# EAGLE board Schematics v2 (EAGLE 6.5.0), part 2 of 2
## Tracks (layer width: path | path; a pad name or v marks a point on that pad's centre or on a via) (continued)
N$201  (via drill 0.5) (continued)
  Bottom 0.813: C117.2 C118.2 23.76,93.34 23.24,93.34 22.73,93.85 v22.73,94.23
N$202
  Top 0.813: C120.1 35.84,91.09 33.53,88.77 19.18,88.77 18.54,88.14 18.54,86.79 U$7.P$6
N$203
  Top 0.813: C121.1 35.84,93.37 32.38,89.92 17.65,89.92 16.64,88.9 16.64,86.67 U$7.P$5
N$204
  Top 0.813: C120.2 38.94,88.29 R41.1
N$205
  Top 0.813: R42.1 36.7,96.19 C121.2
N$206
  Bottom 0.813: X9.1 6.41,88.52 8,90.04 10.79,90.04 12.06,88.77 21.43,88.77 C106.1
N$207
  Top 0.406: U$7.P$30 5.69,97.31 JP8.1
N$208
  Top 0.406: U$7.P$1 9.5,87.59 8.32,88.77 7.62,88.77 6.99,89.41 6.99,94.11 6.03,95.06 4.13,95.06 2.98,96.2 2.98,97.09 JP8.2
N$209
  Bottom 0.813: X9.3 6.03,93.6 7.62,92.33 11.81,92.33 12.32,91.82 21.46,91.82 C105.1
N$210
  Bottom 0.813: U$7.P$29 11.28,95.46 L7.1
N$211
  Bottom 0.813: C122.2 63.27,8.48 62.1,9.65 62.1,10.92 61.34,11.68 60.83,11.68 60.33,12.19 60.33,13.54 U$8.P$11 U$8.P$12 U$8.P$13 U$8.P$14
N$212
  Bottom 0.813: C123.2 63.79,13.45 U$8.P$9 | U$8.P$7 U$8.P$8 U$8.P$9 | U$8.P$9 U$8.P$10
N$213
  Bottom 0.813: C124.1 54.14,11.39 53.21,12.32 U$8.P$15
N$214
  Bottom 0.813: U$8.P$16 53.24,4.34 53.98,5.08 53.98,8.6 C124.2
N$215
  Bottom 0.813: U$8.P$17 55.02,4.47 55.24,4.7 55.24,8 55.63,8.38 55.88,8.38 56.26,8.76 56.26,11.05 56.64,11.43 58.61,11.43 C125.1
N$216
  Bottom 0.813: C125.2 57.9,9.64 57.4,9.14 57.4,8.38 56.64,7.62 56.64,3.05 U$8.P$18
N$217
  Bottom 0.813: U$8.P$27 72.8,4.79 C126.1
N$218
  Bottom 0.813: U$8.P$26 71.02,5.07 C127.1
N$219
  Bottom 0.813: U$8.P$25 69.24,5.07 C128.1
N$220
  Bottom 0.813: U$8.P$23 65.68,5.07 C129.1
N$221
  Bottom 0.813: U$8.P$24 67.46,5.07 C130.1
N$222
  Bottom 0.813: U$8.P$28 74.57,5.04 C131.1
N$223
  Bottom 0.813: U$8.P$19 58.57,5.07 C132.1
N$224
  Bottom 0.813: U$8.P$20 60.35,5.07 C133.1
N$225
  Bottom 0.813: U$8.P$21 62.13,5.07 C134.1
N$226
  Bottom 0.813: U$8.P$22 63.91,5.07 C135.1
N$227  (via drill 0.5)
  Top 0.813: C136.1 81.05,13.43 v80.42,12.8 | v77.37,11.4 76.33,12.45 U$8.P$2
  Bottom 0.813: v80.42,12.8 79.5,11.81 79.1,11.4 v77.37,11.4
N$228  (via drill 0.5)
  Top 0.813: R43.1 70.77,7.28 v72.01,5.97
  Bottom 0.813: C128.2 C127.2 70.98,6.86 71.5,6.86 71.88,6.48 v72.01,5.97
N$229  (via drill 0.5)
  Top 0.813: R44.1 67.15,7.28 v68.45,5.97
  Bottom 0.813: C129.2 C130.2 67.42,6.86 67.94,6.86 68.45,6.35 v68.45,5.97
N$230  (via drill 0.5)
  Top 0.813: v61.34,6.03 60.33,7.11 59.75,7.11 R45.2
  Bottom 0.813: C133.2 C132.2 60.57,6.87 v61.34,6.03
N$231  (via drill 0.5)
  Top 0.813: R46.2 63.59,7.28 v64.9,5.97
  Bottom 0.813: C134.2 C135.2 63.87,6.86 64.39,6.86 64.9,6.35 v64.9,5.97
N$232
  Top 0.813: C137.1 51.79,9.12 54.1,11.43 68.45,11.43 69.09,12.06 69.09,13.41 U$8.P$6
N$233
  Top 0.813: C138.1 51.79,6.84 55.24,10.29 69.98,10.29 70.99,11.3 70.99,13.54 U$8.P$5
N$234
  Top 0.813: C137.2 50.47,11.92 R47.1
N$235
  Top 0.813: R48.1 50.93,4.01 C138.2
N$236
  Bottom 0.813: X10.1 81.22,11.68 79.63,10.16 76.83,10.16 75.56,11.43 66.2,11.43 C123.1
N$237
  Top 0.406: U$8.P$30 81.94,2.9 JP9.1
N$238
  Top 0.406: U$8.P$1 78.13,12.61 79.31,11.43 80.01,11.43 80.64,10.79 80.64,6.1 81.6,5.14 83.5,5.14 84.64,4 84.64,3.11 JP9.2
N$239
  Bottom 0.813: X10.3 81.6,6.6 80.01,7.87 75.82,7.87 75.31,8.38 66.17,8.38 C122.1
N$240
  Bottom 0.813: U$8.P$29 76.35,4.74 L8.1
N$241  (via drill 0.5)
  Top 0.61: IC2.1 82.8,41.91 82.17,41.27 v81.03,41.27 | 78.28,46.79 78.28,47.19 77.98,47.5 | v77.6,44.83 77.6,46.23 78.22,46.85
  Top 1.016: C140.2 77.98,47.5 77.98,47.09 78.22,46.85 78.28,46.79 R50.2
  Bottom 0.61: v81.03,41.27 80.26,41.27 78.36,43.18 78.36,44.07 v77.6,44.83
N$242
  Bottom 0.61: IC5.2 IC5.1 87.12,85.79 C192.1
N$243
  Bottom 0.61: C193.1 84.84,83.57 84.07,82.8 IC5.6 IC5.7
N$244  (via drill 0.5)
  Top 0.406: IC2.7 81.53,36.47 R51.2
  Top 0.61: IC2.7 81.53,36.32 82.17,35.69 v82.17,34.04 | v73.15,51.05 73.15,51.31 72.01,52.45 72.01,63.63 72.64,64.26 72.64,65.53 73.28,66.17 77.47,66.17 C142.2
  Bottom 0.61: v82.17,34.04 82.17,39.37 81.66,39.88 81.66,40.39 82.04,40.77 82.04,45.47 81.41,46.1 79.12,46.1 76.83,48.39 73.79,48.39 73.15,49.02 v73.15,51.05
N$245
  Top 0.406: U$10.1 78.61,52.45 C140.1
N$246
  Top 0.61: U$10.8 78.61,62.23 C142.1
N$247
  Top 0.406: U$10.2 79.88,52.58 C141.1
N$248
  Top 0.61: U$10.7 79.88,62.35 C143.1
N$249
  Bottom 0.305: U3.3 43.33,53.09 R52.2
N$250  (via drill 0.5)
  Top 0.254: RN2.5 76.74,26.57 77.32,27.15 77.32,29.18 77.06,29.44 74.02,29.44 73.51,28.93 73.51,27.41 73.25,27.15 71.98,27.15 71.22,26.39 70.46,26.39 69.95,25.88 52.68,25.88 JP1.2
  Top 0.305: v78.03,24.61 77.16,24.61 RN2.5
  Bottom 0.305: U1.20 78.28,24.56 v78.03,24.61
N$251  (via drill 0.5)
  Top 0.254: 76.05,25.14 76.05,26.77 76.43,27.15 v76.43,28.55 76.05,28.93 74.27,28.93 74.02,28.68 74.02,26.9 73.76,26.64 72.24,26.64 71.48,25.88 70.71,25.88 70.21,25.38 53.44,25.38 52.43,24.36 JP1.4
  Top 0.305: 76.05,25.14 RN2.6
  Bottom 0.254: U1.18 76.99,27.99 v76.43,28.55
N$252  (via drill 0.5)
  Top 0.254: v74.85,27.94 74.85,26.14 | 74.85,26.14 75.16,25.83 75.16,25.27 RN2.7 | 74.85,26.14 72.49,26.14 71.73,25.38 70.97,25.38 70.46,24.87 55.98,24.87 54.97,23.85 JP1.6
  Bottom 0.254: U1.16 75.69,27.08 v74.85,27.94
N$253  (via drill 0.5)
  Top 0.254: RN2.8 73.92,24.61 v72.24,24.61 71.48,24.61 71.22,24.36 58.01,24.36 57.51,23.85 JP1.8
  Bottom 0.254: U1.14 74.4,25.25 74.02,24.87 72.49,24.87 v72.24,24.61
N$254  (via drill 0.5)
  Top 0.254: JP1.10 61.32,21.82 61.32,19.28 62.08,18.52 68.94,18.52 69.57,19.15 70.84,19.15 71.22,19.53 72.24,19.53 72.75,20.04 v72.75,20.8 73.09,21.14 RN1.5
  Bottom 0.254: U1.11 74.4,21.18 74.02,21.57 73.51,21.57 v72.75,20.8
N$255  (via drill 0.5)
  Top 0.254: RN1.6 75.29,21.04 75.29,20.55 75.54,20.3 75.54,20.04 76.05,19.53 v76.05,18.44 75.39,17.75 70.08,17.75 69.06,16.74 64.62,16.74 v63.86,17.5 | JP1.12 62.59,22.58 63.86,21.31 v63.86,19.41
  Bottom 0.254: v63.86,19.41 v63.86,17.5 | U1.9 75.69,19.25 76.05,18.9
  Bottom 0.305: 76.05,18.9 v76.05,18.44
N$256  (via drill 0.5)
  Top 0.254: v77.6,17.78 77.6,18.75 76.05,20.55 76.05,21 RN1.7 | JP1.14 65.13,22.84 66.37,21.59 71.25,21.59 72.11,22.45 v72.11,22.84
  Bottom 0.254: v72.11,22.84 72.87,22.07 76.56,22.07 | 77.06,20.24 U1.7 | 76.81,21.57 77.06,21.31 77.06,20.24 | 77.06,20.24 77.06,19.35 77.49,18.87 77.49,17.86
  Bottom 0.305: 76.56,22.07 76.81,21.82 76.81,21.57 | 77.49,17.86 v77.6,17.78
N$257
  Bottom 1.016: C192.2 87.12,95.25 X11.1
N$258  (via drill 0.5)
  Top 0.406: v47.24,48.26 v47.24,52.45
  Bottom 0.305: v47.24,52.45 U3.2
  Bottom 0.406: JMP5.2 v47.24,48.26
N$259  (via drill 0.5)
  Top 0.254: JP1.16 67.67,22.84 68.45,22.05 70.81,22.05 71.25,22.48 71.25,23.24 71.73,23.72 72.49,23.72 v73.25,22.96 | RN1.8 77.63,21.14 v78.05,21.57
  Bottom 0.254: v73.25,22.96 73.89,22.96 74.02,22.84 76.56,22.84
  Bottom 0.305: 76.56,22.84 77.8,21.57 v78.05,21.57 78.28,21.26 U1.5
N$260  (via drill 0.5)
  Top 0.406: 50.8,53.09 50.8,48.26 51.56,47.62 51.56,46.48 50.93,45.85 48.13,45.85 47.24,44.96 v47.24,44.7
  Top 0.61: 50.8,53.09 v49.78,53.98
  Bottom 0.406: U3.21 50.06,53.75 v49.78,53.98 | v47.24,44.7 JMP6.2
N$261
  Bottom 0.305: JMP4.2 47.24,51.18 46.61,51.82 45.49,51.82
  Bottom 0.406: 45.49,51.82 U3.1
N$262
  Top 0.61: IC3.2 49.28,36.83 | IC3.5 49.53,40.64 49.28,40.39 49.28,36.83 | 49.28,36.83 48.77,36.32 46.99,36.32 46.61,36.7 46.61,37.59 46.1,38.1 IC3.14
N$263  (via drill 0.5)
  Top 0.406: v83.19,86.61 83.44,86.61 85.98,84.07 89.79,84.07 v90.42,83.44 | v85.72,79.76 85.72,79.25 85.98,78.99 U2.13
  Bottom 0.406: R57.2 73.05,88.42 73.66,89.03 77.72,89.03 80.39,86.36 82.93,86.36 v83.19,86.61 | v90.42,83.44 90.42,81.92 88.9,80.39 86.36,80.39 v85.72,79.76
N$264  (via drill 0.6)
  Top 0.813: v50.67,95.38 43.05,95.38 42.42,94.74 42.42,79.76 42.93,79.25 42.93,65.79 41.66,64.52 41.66,38.1 42.93,36.83 IC3.15
  Bottom 0.61: C144.1 51.56,96.27
  Bottom 0.813: 51.56,96.27 v50.67,95.38
N$265  (via drill 0.6)
  Top 0.813: IC3.4 52.2,39.37 v52.96,40.26 | v51.56,32 v41.4,32
  Bottom 0.61: 43.05,95.38 43.43,95.38 C145.1
  Bottom 0.813: v52.96,40.26 52.58,39.88 52.58,33.02 v51.56,32 | v41.4,32 41.66,32.26 41.66,64.52 43.69,66.55 43.69,89.66 42.42,90.93 42.42,94.74 43.05,95.38
N$268
  Bottom 1.27: C148.1 59.05,95.76 U$9.P$25
N$269
  Bottom 1.27: R58.1 46.89,75.03 U$11.6
N$270
  Bottom 1.27: C149.1 U$9.P$1
N$271
  Bottom 1.27: C150.1 74.68,39.24 U$9.P$2
N$272
  Bottom 1.27: C151.1 U$9.P$5
N$273
  Bottom 1.016: R59.1 77.85,60.18 C152.1 78.11,57.78 78.11,50.93 76.83,49.66 U$9.P$6
N$274
  Bottom 1.016: U$9.P$14 77.5,69.98 R61.2
N$275  (via drill 0.5)
  Top 0.254: v81.69,19.91 81.25,19.48 81.25,18.52 81.64,18.14 JMP1.2
  Bottom 0.254: U1.1 80.9,19.51 80.87,19.91 81.13,19.91
  Bottom 0.305: 81.13,19.91 v81.69,19.91
N$276  (via drill 0.5)
  Top 0.254: v82.22,18.9 82.53,19.23 82.53,20.42 82.14,20.8
  Top 0.305: 82.14,20.8 82.14,21.06 JMP2.2
  Bottom 0.254: U1.2 80.24,19.15 80.62,18.77 82.14,18.77
  Bottom 0.305: 82.14,18.77 v82.22,18.9
N$277  (via drill 0.5)
  Top 0.305: v81.64,27.41 JMP3.2
  Bottom 0.305: U1.21 78.94,27.25 79.1,27.41 v81.64,27.41
N$278
  Bottom 1.016: R60.1 77.83,62.38 C153.1 U$9.P$11
N$279
  Bottom 1.016: C193.2 84.84,90.93 81.92,93.85 X11.3
N$281
  Bottom 1.016: C156.2 R62.2 82.95,65.3 C154.1 81.44,65.28 R60.2
N$282
  Bottom 1.016: R61.1 78.59,66.78 79.38,67.56 C156.1
N$283
  Bottom 0.61: C157.1 74.41,92.19 U$9.P$23
  Bottom 1.016: C187.- 81.92,89.92 78.99,92.84 U$9.P$23
N$284  (via drill 0.5)
  Top 0.406: v62.74,85.22 62.74,88.9 v62.99,89.15
  Bottom 0.406: U$9.P$29 v62.74,85.22 | v62.99,89.15 63.37,89.15 63.75,88.77 63.75,87.77 C158.2
N$285
  Bottom 0.406: C158.1 U$9.P$28
N$286
  Bottom 1.016: U$9.P$31 61.85,80.14 C160.1
N$287
  Bottom 1.016: U$9.P$32 62.1,77.6 C160.2
N$288
  Bottom 0.305: U1.3 79.6,18.11 R49.2
N$289
  Bottom 0.61: U$9.P$33 60.71,75.06 61.09,74.68 62.1,74.68 63.12,73.66 63.12,72.38 C159.1
N$290
  Bottom 0.61: U$9.P$34 61.23,72.52 C159.2
N$291
  Bottom 1.016: U$9.P$35 61.85,69.98 C161.1 62.22,69.71 62.74,70.23 64.37,70.23 R63.1
N$292
  Bottom 1.016: C161.2 62.1,67.94 61.59,67.44 59.44,67.43 U$9.P$36
N$293
  Bottom 1.016: C162.2 62.1,57.78 61.59,57.28 59.44,57.27 U$9.P$40
N$294
  Bottom 1.016: U$9.P$39 61.85,59.82 C162.1 62.1,59.56 62.61,60.07 64.37,60.07 R64.1
N$295
  Top 1.016: U$9.P$41 C163.2
  Bottom 1.016: R65.1 59.59,54.89 U$9.P$41
N$296
  Bottom 1.016: U$9.P$46 C166.2
N$297
  Top 1.016: U$9.P$42 C170.2
N$298
  Bottom 1.016: U$9.P$43 C169.2
N$299
  Bottom 1.016: U$9.P$44 C168.2
N$300
  Bottom 1.016: U$9.P$45 C167.2
N$301
  Bottom 1.016: U$9.P$47 C165.2
N$302
  Bottom 1.016: U$9.P$48 C164.2
N$303
  Bottom 1.016: R65.2 66.17,52.05 | 66.17,52.05 66.55,52.05 R66.1 66.53,52.07 | C171.2 66.15,52.06 66.17,52.05
N$304
  Bottom 1.016: C171.1 R64.2 66.14,57.25 66.17,57.28 66.55,57.28 C172.2
N$305
  Top 1.27: U$9.P$37 C173.2
  Bottom 1.016: U$9.P$37 61.82,64.9 R67.1
N$306
  Bottom 1.016: R67.2 64.37,62.33 C174.2 64.39,62.74 64.77,62.36 66.53,62.35 R68.1
N$307
  Bottom 1.016: C174.1 R63.2 65.94,67.41 C175.2
N$308
  Bottom 1.016: C176.2 R69.2
N$309
  Top 1.016: R71.1 57.05,85.06 57.15,84.96 54.48,84.96 U$11.15
  Bottom 0.61: C177.1 54.23,85.21 U$11.15
N$310
  Bottom 1.016: C178.2 54.1,69.59 U$11.9
N$311
  Bottom 1.27: U$11.11 51.82,74.93 C179.2
N$312
  Bottom 1.27: U$11.10 51.69,72.39 C178.1
N$313
  Top 1.27: R72.2 54.99,76.83 54.38,77.44 54.38,77.5 U$11.12
  Bottom 1.27: U$11.12 51.82,77.47 C179.1
N$314  (via drill 0.5)
  Top 0.813: R72.1 v56.9,72.52 C180.1
  Bottom 0.813: v56.9,72.52 56.9,67.56 C181.1
N$315
  Bottom 1.27: U$11.7 49.4,72.39 C183.1
N$316
  Bottom 1.27: U$11.8 46.74,67.94 47.37,67.31 C182.1
N$317
  Bottom 1.016: U$11.2 46.99,85.09 C185.1
N$318
  Top 0.406: U$10.4 82.42,52.22 R53.2
  Top 0.61: JP13.2 85.09,52.7 84.45,52.07 82.83,52.07 R53.2
N$319
  Top 0.61: R54.1 82.42,62.46 U$10.5 83.54,60.48 JP13.1
N$320
  Top 0.406: R56.2 90.93,68.83 91.69,69.6 91.69,80.39 90.55,81.53 U2.15
  Top 0.813: R56.2 89.56,68.68 91.06,67.31 91.06,63.12 89.92,61.98 JP14.2
N$321
  Top 0.406: R55.2 89.28,71.37 | 89.28,71.37 88.14,70.23 88.14,65.15 JP14.1 | 89.28,71.37 89.28,72.01 90.68,73.41 90.68,79.63 90.04,80.26 U2.14
RFED
  Top 0.61: C143.2 80.39,64.52 80.14,64.26 76.83,64.26 76.2,63.63 73.66,63.63 73.03,62.99 73.03,60.45 73.66,59.82 U$9.P$10
RLOUT
  Bottom 1.27: X15.4 49.02,96.9 C144.2
RMIX  (via drill 0.5)
  Top 0.406: IC2.6 80.26,36.73 R51.1
  Top 0.813: R42.2 38.86,97.54 38.23,98.17 v36.83,98.17 | v37.21,13.97 38.51,13.97 R6.2 39.01,13.46 39.75,13.46 42.19,11.02 X6.1 43.94,11.05 44.7,11.05 48.67,7.09 R48.2 | R12.2 38.86,28.32 38.23,28.96 v37.21,28.96 | R18.2 37.85,42.29 v37.21,42.93 | R36.2 38.61,83.82 v37.21,85.22 | R30.2 37.97,69.98 v37.21,70.74 | R24.2 38.48,56.01 v37.21,57.28 | R51.1 79.38,34.67 78.87,34.04 76.71,34.04 74.8,32.13 71.25,32.13 v67.18,28.07
  Bottom 0.813: v36.83,98.17 36.83,89.41 37.21,89.03 v37.21,85.22 v37.21,70.74 v37.21,57.28 v37.21,42.93 v37.21,28.96 37.21,21.21 | 37.21,21.21 38.99,19.43 X14.1 44.07,19.3 44.7,19.3 46.99,21.59 46.99,23.11 50.93,27.05 66.17,27.05 v67.18,28.07 | 37.21,21.21 v37.21,13.97
RO1  (via drill 0.5)
  Top 0.61: v66.29,92.84 U$9.P$26
  Top 0.813: IC3.3 52.2,38.1 55.63,34.67 60.96,34.67 61.98,35.69 61.98,80.64 62.87,81.53 62.87,83.31 61.59,84.58 v61.59,89.15
  Bottom 0.61: C147.1 56.77,90.17 U$9.P$26 60.2,92.84 | IC5.3 88.27,82.8 88.9,83.44 88.9,96.52 87.76,97.66 74.42,97.66 69.6,92.84 v66.29,92.84
  Bottom 0.813: v61.59,89.15 61.59,91.44 60.2,92.84
ROUT
  Bottom 1.016: X15.2 54.1,90.17 C147.2
RROUT
  Bottom 1.27: X15.5 C145.2
RT
  Bottom 1.016: U$9.P$7 74.8,52.2 69.85,57.15 C172.1
SC0  (via drill 0.5)
  Top 0.406: v48.26,57.66 45.59,57.66 43.94,59.31 JP12.1
  Bottom 0.305: U3.5 47.04,54.41 48.01,55.37 48.01,57.78
  Bottom 0.406: 48.01,57.78 v48.26,57.66
SC1
  Bottom 0.305: U3.7 46.56,55.7 46.74,55.88 46.74,59.44 46.48,59.69 45.59,59.69 45.21,60.07 45.21,62.23 JP12.3
SCL
  Bottom 0.254: JP1.18 70.84,23.72 72.62,23.72 73.25,24.36 76.81,24.36
  Bottom 0.305: 76.81,24.36 77.44,23.72 78.46,23.72 79.6,24.87 U1.22
SCLL  (via drill 0.5)
  Top 0.305: v52.2,59.94 51.94,59.69 49.15,59.69 48.39,60.45 v48.39,61.59
  Bottom 0.305: U3.22 52.07,53.09 52.45,53.47 52.45,59.69 v52.2,59.94 | v48.39,61.59 48.39,62.36 49.53,63.5 JP11.2
SD0
  Bottom 0.254: U1.4 78.94,17.09 78.33,16.48 72.98,16.48 | RN3.4 72.91,15.89 72.49,15.47 69.7,15.47 67.67,17.5 JP1.15
  Bottom 0.305: 72.98,16.48 RN3.4
SD1  (via drill 0.5)
  Top 0.254: v66.4,19.41 v68.56,19.41
  Bottom 0.254: v66.4,19.41 JP1.13 | v68.56,19.41 68.94,19.02 68.94,16.99 69.98,15.95 72.03,15.95 72.24,16.15 72.24,16.99 72.6,17.36 RN3.3 73.02,17.25 73.25,17.25 73.51,16.99 78.08,16.99 78.41,17.32 78.41,18.69 77.57,19.53 77.57,20.09 U1.6
SD2
  Bottom 0.254: JP1.11 63.63,21.59 68.91,21.59 69.06,21.44 69.06,20.17 69.83,19.41 70.71,19.41 70.87,19.56 72.24,19.56 72.24,18.26 72.35,18.16 RN3.2 73.02,18.01 73.25,18.01 73.79,17.48 76.56,17.48 76.81,17.75 76.81,18.11 76.99,18.29 76.99,18.72 76.35,19.36 U1.8
SD3
  Bottom 0.254: U1.10 75.03,19.28 75.26,19.05 75.26,18.16 75.11,18.01 74.02,18.01 73.64,18.39 73.64,18.52 73.38,18.77 73.1,18.77 RN3.1 | 73,19.02 72.98,19.02 RN3.1 | RN3.1 72.91,19.62 72.49,20.04 71.48,20.04 71.35,20.17 71.35,21.18 70.46,22.05 60.78,22.05 60.05,21.31 JP1.9
SD4
  Bottom 0.254: U1.13 73.74,26.92 73.25,27.41 72.73,27.41 | RN4.4 72.66,26.3 70.97,24.61 59.28,24.61 58.78,24.11 58.78,21.57 58.01,20.8 57.76,20.8 JP1.7
  Bottom 0.305: 72.73,27.41 RN4.4
SD5
  Bottom 0.254: U1.15 75.03,26.9 74.78,27.15 74.27,27.15 73.25,28.17 72.77,28.17 | RN4.3 72.09,28.28 71.98,28.17 71.98,26.39 70.71,25.12 57,25.12 56.24,24.36 56.24,21.82 JP1.5
  Bottom 0.305: 72.77,28.17 RN4.3
SD6
  Bottom 0.254: U1.17 76.3,27.53 75.64,28.19 75.64,28.45 74.91,29.18 72.77,29.18 | 72.35,29.08 71.98,29.44 71.98,30.25 71.75,30.48 70.74,30.48 70.46,30.2 70.46,28.68 69.52,27.76 69.52,26.47 68.68,25.63 55.73,25.63 54.71,24.61 54.2,24.61 53.7,24.11 53.7,21.82 JP1.3
  Bottom 0.305: 72.77,29.18 RN4.2 72.35,29.08
SD7
  Bottom 0.254: U1.19 77.65,29.36 77.06,29.95 72.73,29.95 | 72.66,30.29 71.98,30.96 70.46,30.96 69.95,30.45 69.95,28.93 69.04,27.99 69.04,26.75 68.43,26.14 52.93,26.14 51.16,24.36 51.16,21.82 JP1.1
  Bottom 0.305: 72.73,29.95 RN4.1 72.66,30.29
SD8  (via drill 0.5)
  Top 0.305: v49.15,58.55 49.02,58.55 47.5,59.94 JP12.2
  Bottom 0.305: U3.4 47.4,53.75 49.15,55.5 v49.15,58.55
SD9
  Bottom 0.305: U3.6 46.79,55.04 47.37,55.63 47.37,60.2 47.62,60.45 47.62,61.21 47.5,61.34 47.5,62.48 JP12.4
SDA  (via drill 0.5)
  Top 0.254: JP1.17 71.22,20.55 72.49,21.82 77.11,21.82 77.85,22.55 78.05,22.55
  Top 0.305: 78.05,22.55 v78.05,22.84
  Bottom 0.254: U1.23 80.24,24.74
  Bottom 0.305: 80.24,24.74 78.33,22.84 v78.05,22.84
SDAA
  Bottom 0.305: U3.23 50.04,52.45 48.9,53.59 48.9,54.36 49.78,55.24 49.78,57.78 50.04,58.04 50.04,60.58 JP11.1
SFED  (via drill 0.5 pad 0.25)
  Top 0.61: v56.9,78.36 55.88,78.36 55.37,78.74 53.09,78.74 52.32,77.98 52.32,75.56 51.94,75.18 51.94,65.79 52.45,65.28 52.45,63.75 53.47,62.74 53.47,59.05 51.05,56.64 44.7,56.64 42.67,54.61 42.67,41.15 43.18,40.64 IC3.12
  Top 1.016: R70.1 59.41,82.7 U$9.P$30
  Bottom 0.61: U$9.P$30 56.9,80.14 R69.1 v56.9,78.36
V-  (via drill 0.5, 0.6)
  Top 0.61: IC3.7 56.64,43.18 56.77,43.31 | v71.75,50.93 70.99,51.69 70.99,64.39 v71.25,64.64 71.25,65.91 72.77,67.44 U$9.P$13 78.23,67.44 v80.01,69.22 | v69.47,41.02 71.5,41.02 73.79,43.31 78.93,43.31 IC2.4
  Top 0.813: U$9.P$27 65.91,90.3 66.8,89.41 66.8,87.25 67.94,86.11 70.23,86.11 71.12,85.22 71.12,83.69 70.74,83.31 66.29,83.31 65.41,82.42 65.41,79.63 65.28,79.63 64.64,78.99 64.64,66.67 v65.91,65.41 | v54.1,32 54.1,31.37 55.75,29.72 v56.52,29.72
  Top 1.27: C173.1 C163.1 56.65,57.66 56.01,57.66 54.74,56.39 54.74,50.29 55.63,49.4 C170.1 v56.77,43.43 56.77,43.31 | v40.89,30.23 v51.18,30.23
  Bottom 0.61: C151.2 71.75,49.65 v71.75,50.93 | v69.47,41.02 69.59,40.89 C150.2 | v65.91,65.41 70.48,65.41 v71.25,64.64 | IC5.4 85.09,81.53 84.07,80.52 84.07,77.22 84.71,76.58 85.98,76.58 86.61,75.95 86.61,72.9 84.96,71.25 82.3,71.25 81.66,70.61 81.66,69.98 80.9,69.22 v80.01,69.22
  Bottom 0.813: v56.52,29.72 65.53,29.72 69.6,33.78 69.6,34.8 C149.2
  Bottom 1.016: C169.1 C168.1
  Bottom 1.27: C164.1 66.8,36.96 67.18,37.34 C190.2 67.19,36.96 C149.2 C150.2 | C164.1 C165.1 C166.1 C167.1 64.9,46.99 C168.1 C151.2 | C169.1 64.77,47.49 64.9,47.37 64.9,46.99 | C164.1 | v56.77,43.43 56.52,43.18 55.37,43.18 54.74,42.55 54.74,39.88 54.1,39.24 C188.- v54.1,32 52.32,30.23 v51.18,30.23 | JP10.3 42.42,22.99 40.89,24.51 v40.89,30.23
VCC  (via drill 0.5, 0.5 pad 0.2, 0.5 pad 0.25, 0.6)
  Top 0.254: RN1.4 RN1.3 RN1.2 RN1.1 | RN2.3 RN2.2 RN2.1 | v70.31,27.41 71.48,27.41 71.73,27.66 73,27.66 73,29.18 73.76,29.95 77.32,29.95 78.84,28.42 78.84,23.85 | 78.84,17.25 78.84,23.85 | RN2.4 78.67,23.68 78.84,23.85
  Top 0.305: RN1.1 RN2.4 RN2.3 | 78.84,28.42 78.84,28.93 | v70.46,16.74 78.33,16.74 78.84,17.25
  Top 0.406: v78.11,85.47 78.11,85.22
  Top 0.61: v65.41,84.45 68.96,84.45 v69.28,84.77 | IC3.16 43.31,35.56 v43.31,34.67 | 46.99,87.38 U$11.1 | R53.1 v82.8,47.5 | v79.63,29.72 78.84,28.93 | U2.3 U2.2 U2.1 | U2.16 85.47,82.8 v83.57,84.71 83.44,84.58 | 76.96,83.95 76.83,83.95 v73.03,83.95
  Top 0.813: C184.1 44.07,86.49 45.21,87.63 U$11.1 | v51.05,83.19 51.05,83.44 49.28,85.22 49.28,86.74 48.64,87.38 46.99,87.38 | R54.2 84.43,65.68 85.34,64.77 | 85.34,64.77 85.34,61.85 87.63,59.56 87.63,55.63 86.74,54.74 86.74,50.16 84.07,47.5 v82.8,47.5 | 83.44,84.58 83.44,71.88 84.07,71.25 86.59,71.25 R55.1 R56.1 86.72,66.14 85.34,64.77 | U2.1 78.11,82.8 76.96,83.95 | 78.11,85.22 76.83,83.95 | v80.26,40.01 82.8,40.01 v82.93,40.13 82.93,38.29 IC2.8
  Top 1.016: v69.47,42.67 69.47,42.8 71.25,44.58 U$9.P$4 | C189.+ 58.17,29.21 57.15,28.19 52.83,28.19 52.83,33.15 51.82,34.16 43.81,34.16 v43.31,34.67
  Top 1.27: 62.61,31.75 62.48,31.62 58.29,31.62 C189.+ | v69.47,42.67 66.42,42.67 65.66,41.91 65.66,34.8 62.61,31.75 | v89.89,24.36 89.89,29.44 88.37,30.96 80.87,30.96 v79.63,29.72 | 62.61,31.75 68.07,31.75 70.23,33.91 v74.04,33.91
  Bottom 0.254: RN3.5 RN3.6 RN3.7 RN3.8 71.56,17.59 71.22,17.63 70.46,16.87 v70.46,16.74
  Bottom 0.305: RN4.8 RN4.7 RN4.6 RN4.5 70.53,27.48 v70.31,27.41 | C40.1 85.95,20.8 88.49,20.8 90.02,22.33 | 90.02,25.38 90.78,26.01
  Bottom 0.406: 78.23,85.34 v78.11,85.47
  Bottom 0.61: U$11.1 48.39,87.63 49.4,86.61 52.96,86.61 53.21,86.36 55.63,86.36 55.75,86.49 60.83,86.49 60.96,86.61 63.37,86.61 64.01,85.98 64.01,84.96 64.52,84.45 v65.41,84.45 | v80.26,40.01 79.25,40.01 77.34,41.91 77.34,43.43 76.2,44.58 U$9.P$4 | v82.8,47.5 82.8,45.97 82.93,45.85 v82.93,40.13 | JP10.1 43.94,28.32 42.67,29.59 42.67,32.64 43.56,33.53 44.53,33.53 | v73.03,83.95 72.01,83.95 | 72.01,83.95 70.1,83.95 v69.28,84.77 | R57.1 71.88,84.07 72.01,83.95
  Bottom 0.813: C186.1 51.69,82.17 51.05,82.8 v51.05,83.19 | 88.49,20.8 X5.2 | v83.57,84.71 82.93,85.34 IC5.8 78.23,85.34
  Bottom 1.016: C191.1 71.12,42.04 70.48,42.67 v69.47,42.67 | C40.1 85.82,20.8 85.95,20.8 X5.2 | 91.14,22.81 IC1.3 89.89,25.83 v89.89,24.36 | IC4.3 43.92,34.06 v43.31,34.67 43.56,34.42 43.56,33.53
  Bottom 1.27: 91.14,22.81 88.49,20.8 | 90.02,22.33 90.02,25.38 | v74.04,33.91 75.56,33.91 v79.63,29.72

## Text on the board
Top: 8 Channel Mixer / Master Controller
Bottom: Designed by / Sunny Lee | Ver 2.0
tPlace: SCL | SDA | GND | COUT | ROUT | LOUT | RROUT | RLOUT | LPhone | RPhone | SCL | SD1 | SC0 | SC1 | SDA | SC1 | SD1 | SC0 | SD0 | SD0 | LMIX | RMIX | A2 | CAY16 | A1 | 0 1 | SCL | SC7 | A0 | SC6 | SC5 | SC4 | SC3 | SC2 | SC1 | SC0 | 0805 | GND | 5V | SD7 | 9V | SDA | SD0 | RIN | GND | LIN | SCL | SDA
bPlace: A0 | 1 0 | A1 | A2 | 0805 | +5V | GND | CAY16 | -5V | CAY16 | RMIX | LMIX | GND
_tNames: C27 | C28 | C30 | C29 | C35 | C34 | C33 | C32 | C36 | C37 | R11 | X2 | C38 | R12 | C8 | C9 | C11 | C10 | C16 | C15 | C14 | C13 | C39 | IC2 | C17 | C18 | R5 | X1 | C19 | R6 | C40 | X10 | X11 | X9 | X12
_bNames: IC1 | R10 | R9 | C31 | C26 | R7 | R8 | C21 | C25 | C24 | C20 | C22 | R4 | R3 | C23 | C12 | C7 | R1 | R2 | C2 | C1 | C6 | C5 | C4 | C3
